TEXTLIST TextList_Payment
  0 = '激活' | chinese: '激活' | english: 'Active'
  1 = '开始时间--年' | chinese: '开始时间--年' | english: 'Year'
  2 = '开始时间--月' | chinese: '开始时间--月' | english: 'Month'
  3 = '开始时间--日' | chinese: '开始时间--日' | english: 'Day'
  4 = '分期期数' | chinese: '分期期数' | english: 'Payment Time'
  5 = '两期间隔月数' | chinese: '两期间隔月数' | english: 'Interval Month'
  6 = '提前通知天数' | chinese: '提前通知天数' | english: 'Ahead Days'
  9 = '请输入解锁密码' | chinese: '请输入解锁密码' | english: 'Unlock Password'
  10 = '设定' | chinese: '设定' | english: 'Setting'
  11 = '实际' | chinese: '实际' | english: 'Actual'
  100 = '禁用' | chinese: '禁用' | english: 'Disable'
  101 = '启用' | chinese: '启用' | english: 'Enable'
  102 = '提示将要锁机' | chinese: '提示将要锁机' | english: '提示将要锁机'
  103 = '锁机报警' | chinese: '锁机报警' | english: '锁机报警'
  109 = '当前期数' | chinese: '当前期数' | english: '当前期数'
  110 = '说明:' | chinese: '说明:' | english: '说明:'
  111 = '1. 先输入开始计算分期的日期密码等，' | chinese: '1. 先输入开始计算分期的日期密码等，' | english: '1. 先输入开始计算分期的日期密码等，'
  112 = '   然后点击“激活”按钮，开始计时。' | chinese: '   然后点击“激活”按钮，开始计时。' | english: '   然后点击“激活”按钮，开始计时。'
  113 = '2. 激活后，上方的状态切换为“启用”，' | chinese: '2. 激活后，上方的状态切换为“启用”，' | english: '2. 激活后，上方的状态切换为“启用”，'
  114 = '   并显示当前已经到第几期密码。启用' | chinese: '   并显示当前已经到第几期密码。启用' | english: '   并显示当前已经到第几期密码。启用'
  115 = '   后，不能再修改开始日期，如果要修' | chinese: '   后，不能再修改开始日期，如果要修' | english: '   后，不能再修改开始日期，如果要修'
  116 = '   改，只能是输入最后一期密码解锁后，' | chinese: '   改，只能是输入最后一期密码解锁后，' | english: '   改，只能是输入最后一期密码解锁后，'
  117 = '   重新激活。启用后，可以修改各期密\t' | chinese: '   重新激活。启用后，可以修改各期密\t' | english: '   重新激活。启用后，可以修改各期密\t'
  118 = '   码，修改后再按下“激活”按钮生效。' | chinese: '   码，修改后再按下“激活”按钮生效。' | english: '   码，修改后再按下“激活”按钮生效。'
  119 = '3. 密码不能设置成一样，否则只是最低等' | chinese: '3. 密码不能设置成一样，否则只是最低等' | english: '3. 密码不能设置成一样，否则只是最低等'
  120 = '   级的有效，密码不能设置成"9999999"' | chinese: '   级的有效，密码不能设置成"9999999"' | english: '   级的有效，密码不能设置成"9999999"'
  121 = ''
  122 = ''
  123 = ''
  124 = ''
  125 = ''
   = ''
END_TEXTLIST
